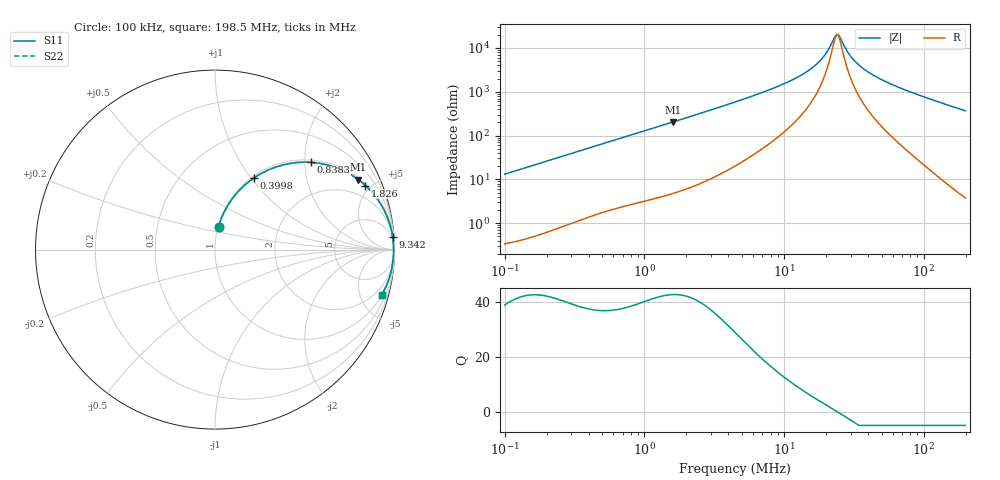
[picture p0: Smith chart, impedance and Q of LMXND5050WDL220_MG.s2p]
! LMXND5050WDL220_MG  S-PARAMETER MODEL  ( General Type )
! Model Generated by TAIYO YUDEN Corporation (https://www.yuden.co.jp/en/)
! Version 1.0
! TAIYO YUDEN Control No. 191023NI43SB-FBB
! Copyright(c) 2019 TAIYO YUDEN CO.,LTD. All Rights Reserved.
! Product Description (link to TY-COMPAS)
! https://ds.yuden.co.jp/TYCOMPAS/or/detail?pn=LMXND5050WDL220MMG&u=M
! Products Name : Inductors
! Characteristics :
!  Inductance : 22 uH , SRF(min) : 15 MHz , DC Resistance(max) : 0.276 Ohm
!  Rated Current : Saturation :1200 mA , Temp Rise : 820 mA (40 degC)
!  Case Size : 4.9 x 4.9 / 0.193 x 0.193 [mm/inch] , Thickness : 2.4 / 0.094 [mm/inch]
!  (Conditions: Temperature = 25 degC , DC Bias Current/Voltage = 0A / 0V)
! External Node Assignments :
!  1  o---GGG---o  2
! GND o---------o GND
! Frequency Range : 0.1MHz  -  198.534594MHz  [ 402 STEP ]
# MHz S RI R 50
! Freq[MHz].  S11 Real  S11 Imag  S21 Real  S21 Imag  S12 Real  S12 Imag  S22 Real  S22 Imag
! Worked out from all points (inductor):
!   401 points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, 100 kHz to 198.5 MHz, reference 50 ohm
!   read as one part in series: L = 20.8 uH near 103.9 kHz
!   highest Q = 42.7 at 1.598 MHz (marker M1), where L = 20.2 uH
!   self-resonance near 23.68 MHz
!   S11 on the Smith chart (normalised r, x): 100 kHz: 1.01, +0.26; 399.8 kHz: 1.03, +1.03; 838.3 kHz: 1.06, +2.14; 1.826 MHz: 1.11, +4.64; 9.342 MHz: 3, +28; 198.5 MHz: 1.08, -7.33
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0.1  0.0201 0.1281  0.9799 -0.1281  0.9799 -0.1281  0.0201 0.1281
0.205728  0.0725 0.2476  0.9275 -0.2476  0.9275 -0.2476  0.0725 0.2476
0.356769  0.1826 0.3735  0.8174 -0.3735  0.8174 -0.3735  0.1826 0.3735
0.399811  0.2173 0.3993  0.7827 -0.3993  0.7827 -0.3993  0.2173 0.3993
0.83829  0.5331 0.4862  0.4669 -0.4862  0.4669 -0.4862  0.5331 0.4862
1.272844  0.7191 0.4377  0.2809 -0.4377  0.2809 -0.4377  0.7191 0.4377
1.598491  0.7995 0.3888  0.2005 -0.3888  0.2005 -0.3888  0.7995 0.3888
1.82567  0.8378 0.3571  0.1622 -0.3571  0.1622 -0.3571  0.8378 0.3571
4.541117  0.967 0.1618  0.033 -0.1618  0.033 -0.1618  0.967 0.1618
9.342371  0.9897 0.0709  0.0103 -0.0709  0.0103 -0.0709  0.9897 0.0709
12.65816  0.9929 0.0447  0.00711 -0.0447  0.00711 -0.0447  0.9929 0.0447
15.89665  0.9942 0.0278  0.0058 -0.0278  0.0058 -0.0278  0.9942 0.0278
19.21992  0.9948 0.0147  0.0052 -0.0147  0.0052 -0.0147  0.9948 0.0147
22.80095  0.9951 0.00343  0.00494 -0.00343  0.00494 -0.00343  0.9951 0.00343
24.13719  0.9951 -0.000294  0.00491 0.000294  0.00491 0.000294  0.9951 -0.000294
25.07124  0.9951 -0.00278  0.0049 0.00278  0.0049 0.00278  0.9951 -0.00278
29.74248  0.995 -0.0141  0.00503 0.0141  0.00503 0.0141  0.995 -0.0141
33.96951  0.9947 -0.0231  0.0053 0.0231  0.0053 0.0231  0.9947 -0.0231
41.85813  0.9939 -0.0382  0.00611 0.0382  0.00611 0.0382  0.9939 -0.0382
56.71438  0.9916 -0.0634  0.00843 0.0634  0.00843 0.0634  0.9916 -0.0634
98.35271  0.9804 -0.1252  0.0196 0.1252  0.0196 0.1252  0.9804 -0.1252
198.5346  0.9285 -0.2526  0.0715 0.2526  0.0715 0.2526  0.9285 -0.2526
